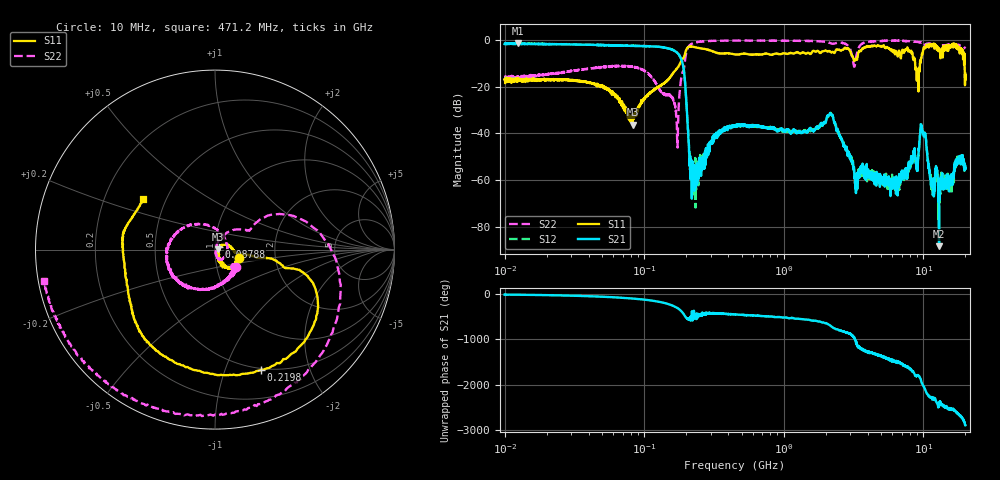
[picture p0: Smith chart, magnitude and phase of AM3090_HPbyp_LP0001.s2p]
# Hz S DB R 50
!freq MagS11 AngS11 MagS21 AngS21 MagS12 AngS12 MagS22 AngS22
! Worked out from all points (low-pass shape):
!   3201 points, 10 MHz to 20 GHz, reference 50 ohm
!   highest |S21| = -1.45 dB at 12.41 MHz (marker M1); lowest = -88.2 dB at 12.95 GHz (marker M2)
!   |S21| within 3 dB of the highest: start of sweep to 161.8 MHz
!   lowest |S11| = -36.3 dB at 82.62 MHz (marker M3), VSWR 1.03, Z = 51.5 + j0.254 ohm
!   |S11| at or under -10 dB: start of sweep to 181 MHz; 8.729 GHz to 9.453 GHz (723.8 MHz wide, 7.96 % of centre); 19.73 GHz to end of sweep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
!   |S22| runs from -46.0 to -0.2 dB; largest |S21 - S12| = 0.03
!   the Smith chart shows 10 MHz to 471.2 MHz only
!   S11 on the Smith chart (normalised r, x): 10 MHz: 1.31, -0.12; 87.88 MHz: 1.05, +0.03; 219.8 MHz: 0.48, -1.34; 471.2 MHz: 0.37, +0.28
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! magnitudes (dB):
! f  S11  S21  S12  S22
! 10 MHz  -16.9  -1.8  -1.6  -16.3
! 12.41 MHz  -17.4  -1.4  -1.7  -16.0
! 35.55 MHz  -17.7  -2.0  -2.0  -12.7
! 82.62 MHz  -36.3  -2.5  -2.5  -11.5
! 87.88 MHz  -31.7  -2.6  -2.5  -11.7
! 126.1 MHz  -20.3  -2.9  -2.9  -20.4
! 170.5 MHz  -12.4  -5.3  -5.2  -34.3
! 186.2 MHz  -8.6  -8.9  -8.9  -14.9
! 219.8 MHz  -2.9  -57.9  -56.2  -1.6
! 447.2 MHz  -6.2  -36.7  -36.6  -0.3
! 471.2 MHz  -6.2  -36.1  -36.5  -0.3
! 1.59 GHz  -5.3  -38.6  -38.3  -0.5
! 2.181 GHz  -5.3  -31.8  -31.6  -1.5
! 3.297 GHz  -8.2  -62.7  -62.9  -7.5
! 5.639 GHz  -3.7  -62.4  -59.3  -0.3
! 7.901 GHz  -4.5  -53.0  -54.6  -0.6
! 9.004 GHz  -15.9  -56.0  -54.9  -0.9
! 9.878 GHz  -5.5  -39.5  -39.5  -1.3
! 11.5 GHz  -2.1  -61.4  -63.9  -2.0
! 12.95 GHz  -3.5  -88.2  -76.5  -2.9
! 17.14 GHz  -2.4  -54.0  -52.7  -2.1
! 20 GHz  -14.5  -55.0  -53.4  -3.7
